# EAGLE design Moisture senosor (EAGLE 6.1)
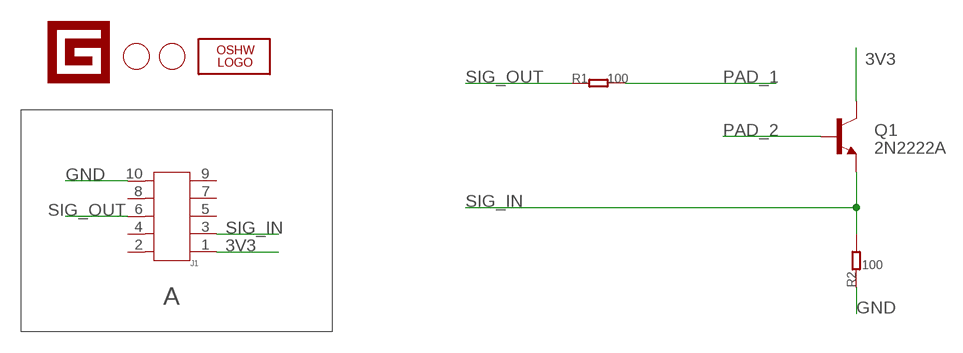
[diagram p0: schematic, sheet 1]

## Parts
J1  HEADER-SHF-105-01-L-D-SM  [SHF-105-01-L-D-SM]
LOGO1  LOGO-OSHW-FILLX0150-NT  [OSHW_FILLX150_NOTEXT]
Q1  2N2222A  TRANSISTOR_NPNTO92  [TO-92]
R1  100  R-0603  [0603]
R2  100  R-0603  [0603]
U$1  LOGO-GADGETEER-NORMAL  [GADGETEER-SILK]
U$2  PAD-HOLE'3.2/7.0'  [HOLE-D-3.2/7.0]
U$3  PAD-HOLE'3.2/7.0'  [HOLE-D-3.2/7.0]

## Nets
3V3: J1.1 Q1.3(C)
GND: J1.10 R2.1
PAD_1: R1.2
PAD_2: Q1.2(B)
SIG_IN: J1.3 Q1.1(E) R2.2
SIG_OUT: J1.6 R1.1
Unconnected: J1.2 J1.4 J1.5 J1.7 J1.8 J1.9

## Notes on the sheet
- A

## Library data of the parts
J1 = Connector:HEADER-SHF-105-01-L-D-SM
LOGO1 = Logo:LOGO-OSHW-FILL
Q1 = SparkFun:TRANSISTOR_NPN: Transistor NPN BJT configuration in SOT23 package. MMBT2222 is the common NPN we use. Double check BCE configuration again layout.
R1 R2 = Discrete:R*
U$1 = Logo:LOGO-GADGETEER
U$2 U$3 = Discreter:PAD-HOLE

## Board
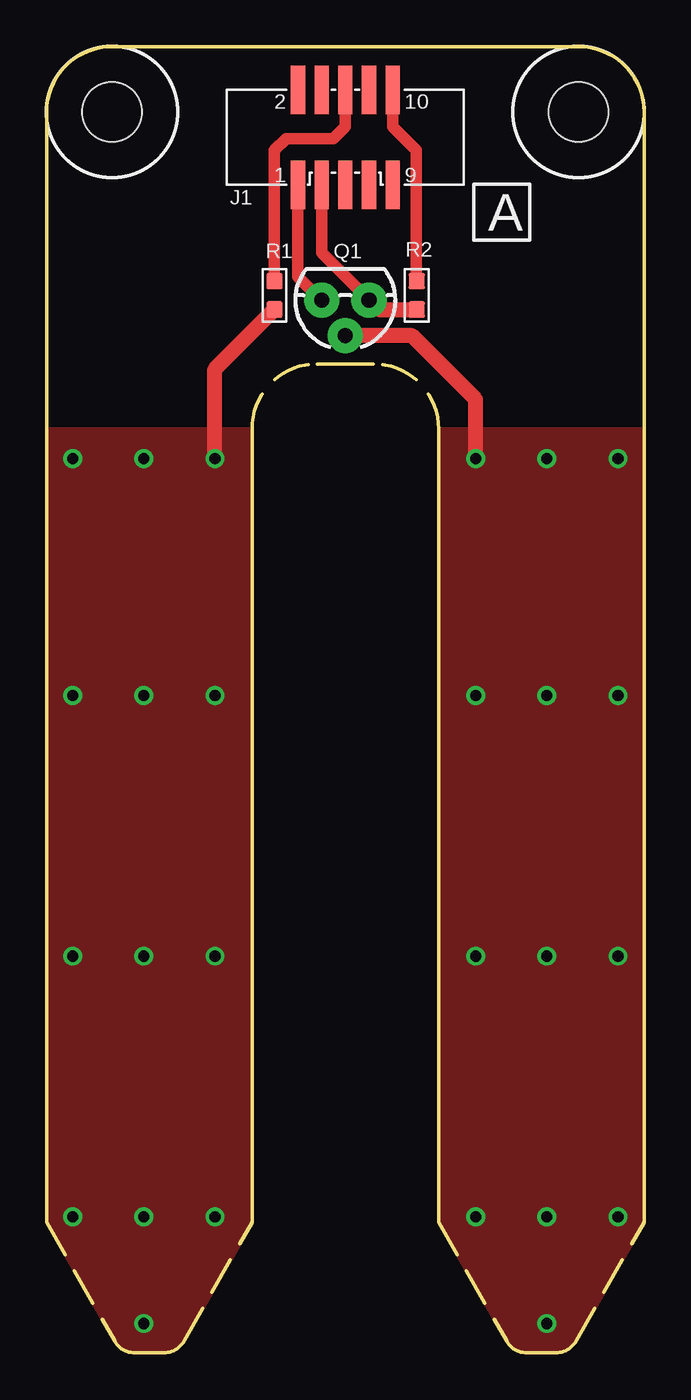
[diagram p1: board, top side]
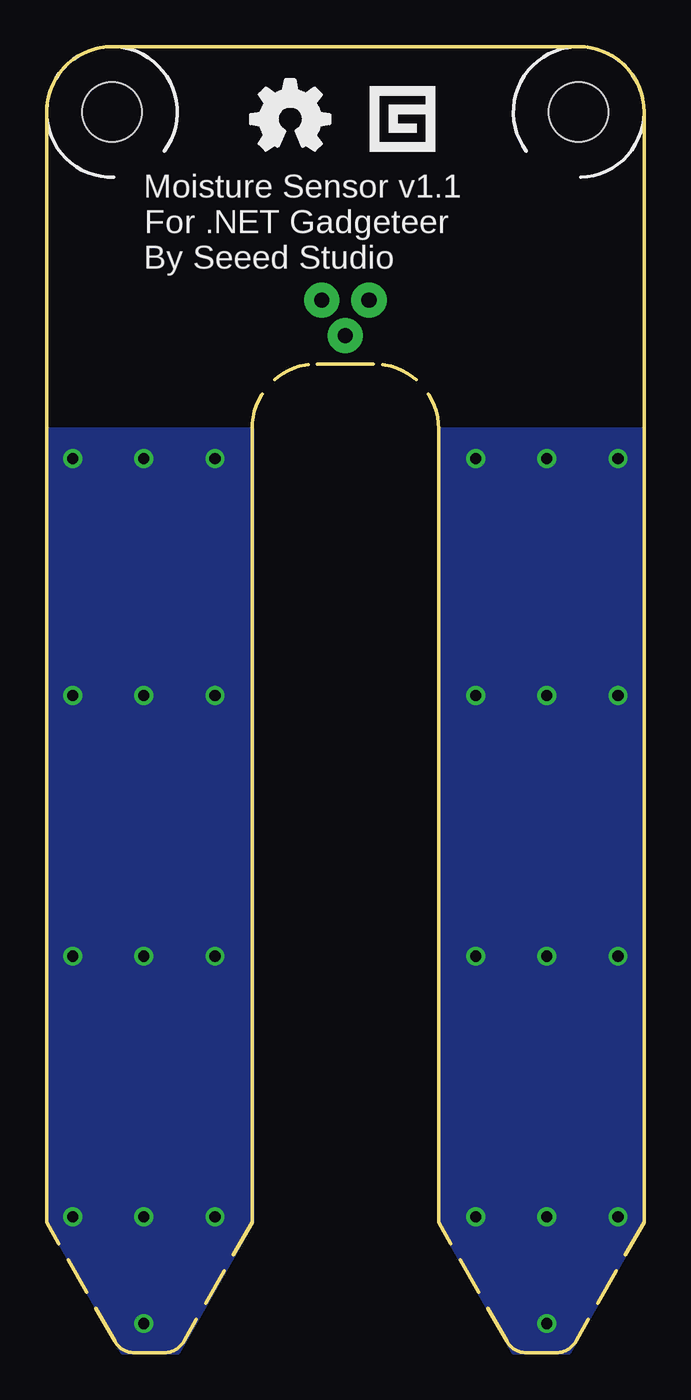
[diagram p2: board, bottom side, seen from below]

Size 32 x 70 mm. Coordinates in mm from the lower left corner, seen from the top.
Outline: 21,7 21,49 21,49.5 arc90 17.5,53 14.5,53 arc90 11,49.5 11,49 11,7 7.37,0.64 arc-60 6.26,0 4.74,0 arc-60 3.63,0.64 0,7 0,66.5 arc-90 3.5,70 28.5,70 arc-90 32,66.5 32,7 28.37,0.64 arc-60 27.26,0 25.74,0 arc-60 24.63,0.64 21,7
Copper layers (1*16): Top 0.035mm / dielectric 1.5mm / Bottom 0.035mm
Design rules: minimum track width 7mil, minimum drill 12mil, track to track 8mil, track to pad 8mil, pad to pad 8mil, via to via 8mil, smd to smd 8mil, copper to edge 0mil, drill to drill 8mil, minimum pad ring 10mil, minimum via ring 8mil, stop-mask expansion 4mil, vias tented up to drill 25mil, thermal gap 10mil

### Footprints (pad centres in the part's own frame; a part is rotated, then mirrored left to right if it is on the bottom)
SHF-105-01-L-D-SM = smd 0.762 x 2.6: 1 -2.54,-2.54; 2 -2.54,2.54; 3 -1.27,-2.54; 4 -1.27,2.54; 5 0,-2.54; 6 0,2.54; 7 1.27,-2.54; 8 1.27,2.54; 9 2.54,-2.546; 10 2.54,2.54
TO-92 = drill 0.813 pad 1.88: 1 -1.27,0; 2 0,1.905; 3 1.27,0
0603 = smd 0.889 x 0.889: 1 -0.762,0; 2 0.762,0
HOLE-D-3.2/7.0 = hole 3.2: 0,0

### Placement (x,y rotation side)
J1  16,65.14 0 top
LOGO1  21.08,64.44 0 bottom
Q1  16,56.42 180 top
R1  12.21,56.67 270 top
R2  19.82,56.67 270 top
U$1  12.52,66.56 0 bottom
U$2  28.5,66.5 0 top
U$3  3.5,66.5 0 top

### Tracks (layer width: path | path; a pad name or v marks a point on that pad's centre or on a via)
3V3
  Top 0.61: J1.1 13.46,57.69 Q1.3
GND
  Top 0.61: J1.10 18.54,65.71 19.81,64.44 19.81,57.45 R2.1
PAD_1  (via drill 0.6)
  Top 0.813: v9.02,47.93 9.02,52.72 R1.2
  other vias: 1.39,7.29 9.02,35.23 9.02,7.29 5.21,35.23 5.21,1.58 5.21,7.29 1.39,35.23 5.21,21.26 1.39,21.26 9.02,21.26 1.39,47.93 5.21,47.93
  pour Top (no thermals): 11,49.5 0,49.5 0,7 3.63,0.64 arc60 4.74,0 6.26,0 arc60 7.37,0.64 11,7
  pour Bottom (no thermals): 11,49.5 0,49.5 0,7.07 arc30 0.03,6.94 4,0 6.5,0 7,0 11,7
PAD_2  (via drill 0.6)
  Top 0.813: v22.98,47.93 22.98,51.11 19.58,54.51 Q1.2
  other vias: 30.61,47.93 22.98,35.23 26.8,35.23 30.61,35.23 22.98,21.26 22.98,7.29 26.8,21.26 26.8,7.29 26.8,1.58 30.61,21.26 30.61,7.29 26.8,47.93
  pour Top (no thermals): 32,49.5 21,49.5 21,7 24.63,0.64 arc60 25.74,0 27.26,0 arc60 28.37,0.64 31.9,6.83 arc15 32,7.07
  pour Bottom (no thermals): 31.95,49.5 20.95,49.5 20.95,7 24.95,0 27.45,0 27.95,0 31.95,7
SIG_IN
  Top 0.61: J1.3 14.73,58.96 Q1.1
  Top 0.813: R2.2 17.78,55.91 Q1.1
SIG_OUT
  Top 0.61: R1.1 12.21,64.45 12.82,65.08 15.37,65.08 16,65.71 J1.6 16,68.25

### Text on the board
tPlace: A
bPlace: Moisture Sensor v1.1 | For .NET Gadgeteer | By Seeed Studio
